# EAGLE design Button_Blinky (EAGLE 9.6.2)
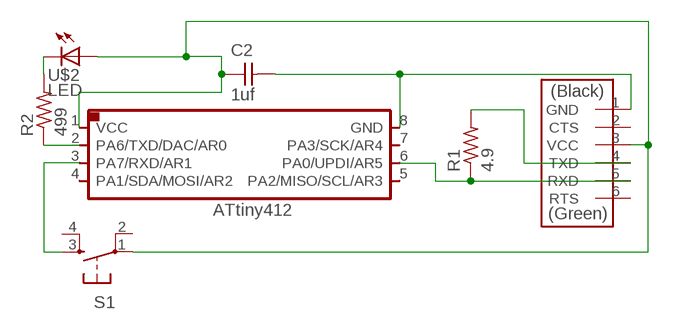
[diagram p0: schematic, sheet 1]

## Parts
C2  1uf  CAP_UNPOLARIZED  [C1206]
R1  4.9  R1206  [R1206]
R2  499  R1206  [R1206]
S1  SW_SWITCH_TACTILE_6MM6MM_SWITCH  [6MM_SWITCH]
U$1  UC_ATTINY412SI  [SOIC8]
U$2  LED  [LED1206]
U$3  CONN_06_FTDI-SMD-HEADER  [1X06SMD]

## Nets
N$1: R1.1 U$1.6(PA0/UPDI/AR5) U$3.5(RXD)
N$2: R1.2 U$3.4(TXD)
N$3: C2.2 U$1.8(GND) U$3.1(GND)
N$4: R2.2 U$2.2(C)
N$5: R2.1 U$1.2(PA6/TXD/DAC/AR0)
N$6: C2.1 S1.1(P) U$1.1(VCC) U$2.1(A) U$3.3(VCC)
N$7: S1.3(S) U$1.3(PA7/RXD/AR1)
Unconnected: S1.2(P1) S1.4(S1) U$1.4(PA1/SDA/MOSI/AR2) U$1.5(PA2/MISO/SCL/AR3) U$1.7(PA3/SCK/AR4) U$3.2(CTS) U$3.6(RTS)

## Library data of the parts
C2 = eagle_fab:CAP_UNPOLARIZED
R1 R2 = eagle_fab:R: Resistor (US Symbol)
S1 = eagle_fab:SW_SWITCH_TACTILE_6MM: OMRON SWITCH
U$1 = fab_new:UC_ATTINY412
U$2 = eagle_fab:LED: LED
U$3 = fab_new:CONN_06_FTDI-SMD-HEADER

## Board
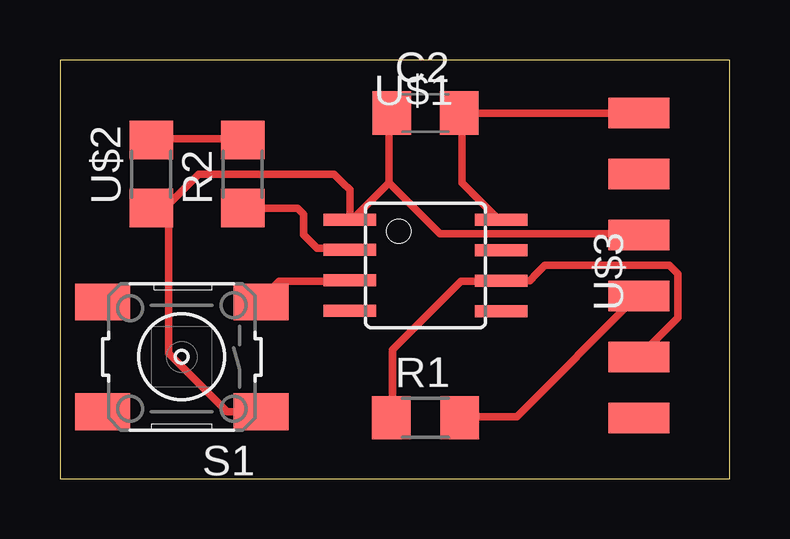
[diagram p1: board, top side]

Size 27.92 x 17.45 mm. Coordinates in mm from the lower left corner, seen from the top.
Outline: 0,0 27.92,0 27.92,17.45 0,17.45 0,0
Copper layers (1*16): Top 0.035mm / dielectric 1.5mm / Bottom 0.035mm
Design rules "OthermillDRC_30_deg_v2": minimum track width 6mil, minimum drill 0.8mm, track to track 6mil, track to pad 6mil, pad to pad 6mil, via to via 6mil, smd to smd 0mil, copper to edge 0mil, drill to drill 6mil, minimum pad ring 10mil, minimum via ring 10mil, stop-mask expansion 1mil, vias tented up to drill 30mil, thermal gap 6mil

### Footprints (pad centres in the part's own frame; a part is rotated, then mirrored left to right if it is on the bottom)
C1206 = smd 1.6 x 1.8: 1 -1.4,0; 2 1.4,0
R1206 = smd 1.6 x 1.803: 1 -1.422,0; 2 1.422,0
6MM_SWITCH = smd 2.286 x 1.524: 1 -3.302,2.286; 2 3.302,2.286; 3 -3.302,-2.286; 4 3.302,-2.286
SOIC8 = smd 0.5 x 2.2: 1 -1.905,-3.154; 2 -0.645,-3.154; 3 0.625,-3.154; 4 1.895,-3.154; 5 1.905,3.154; 6 0.635,3.154; 7 -0.635,3.154; 8 -1.905,3.154
LED1206 = smd 1.6 x 1.803: 1 -1.422,0; 2 1.422,0
1X06SMD = smd 2.54 x 1.27: 1 0,6.35; 2 0,3.81; 3 0,1.27; 4 0,-1.27; 5 0,-3.81; 6 0,-6.35

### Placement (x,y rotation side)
C2  15.24,15.24 0 top
R1  15.24,2.54 0 top
R2  7.62,12.7 90 top
S1  5.08,5.08 180 top
U$1  15.24,8.89 270 top
U$2  3.81,12.7 90 top
U$3  24.13,8.89 0 top

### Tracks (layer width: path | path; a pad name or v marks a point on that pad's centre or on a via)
N$1
  Top 0.152: 13.87,2.59 R1.1 | 18.29,8.23 U$1.6
  Top 0.305: 13.87,2.59 13.87,5.38 16.71,8.23 18.29,8.23 | U$3.5 25.76,6.71 25.76,8.23 25.76,8.53 25.4,8.89 20.22,8.89 19.86,8.53 19.58,8.26 U$1.6
N$2
  Top 0.152: 16.76,2.59 R1.2 | 24.08,7.62 U$3.4
  Top 0.305: 16.76,2.59 19.05,2.59 24.08,7.62
N$3
  Top 0.152: 18.29,10.82 U$1.8 | 16.76,15.24 C2.2
  Top 0.305: 18.29,10.82 16.76,12.34 16.76,15.24 U$3.1
N$4
  Top 0.152: 3.81,14.17 U$2.2 | 7.62,14.17 R2.2
  Top 0.305: 7.62,14.17 3.81,14.17
N$5
  Top 0.152: 11.58,9.6 12.04,9.6 | R2.1
  Top 0.305: R2.1 9.91,11.28 10.16,11.02 10.16,10.16 10.72,9.6 11.58,9.6 | 12.04,9.6 U$1.2
N$6
  Top 0.152: 13.72,15.24 C2.1 | 12.19,10.82 U$1.1 | 3.81,11.43 U$2.1 | 24.08,10.21 U$3.3
  Top 0.305: 13.72,12.34 13.72,15.24 | 12.19,10.82 13.72,12.34 | 4.52,11.43 3.81,11.43 | 4.52,11.43 5.44,12.34 5.79,12.7 11.43,12.7 11.79,12.34 12.09,12.04 U$1.1 | S1.1 6.96,2.79 4.52,5.23 4.52,11.43 | 24.08,10.21 15.85,10.21 13.72,12.34
N$7
  Top 0.152: 12.04,8.23 U$1.3 | 8.38,7.47 S1.3
  Top 0.305: 12.04,8.23 9.14,8.23 8.38,7.47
